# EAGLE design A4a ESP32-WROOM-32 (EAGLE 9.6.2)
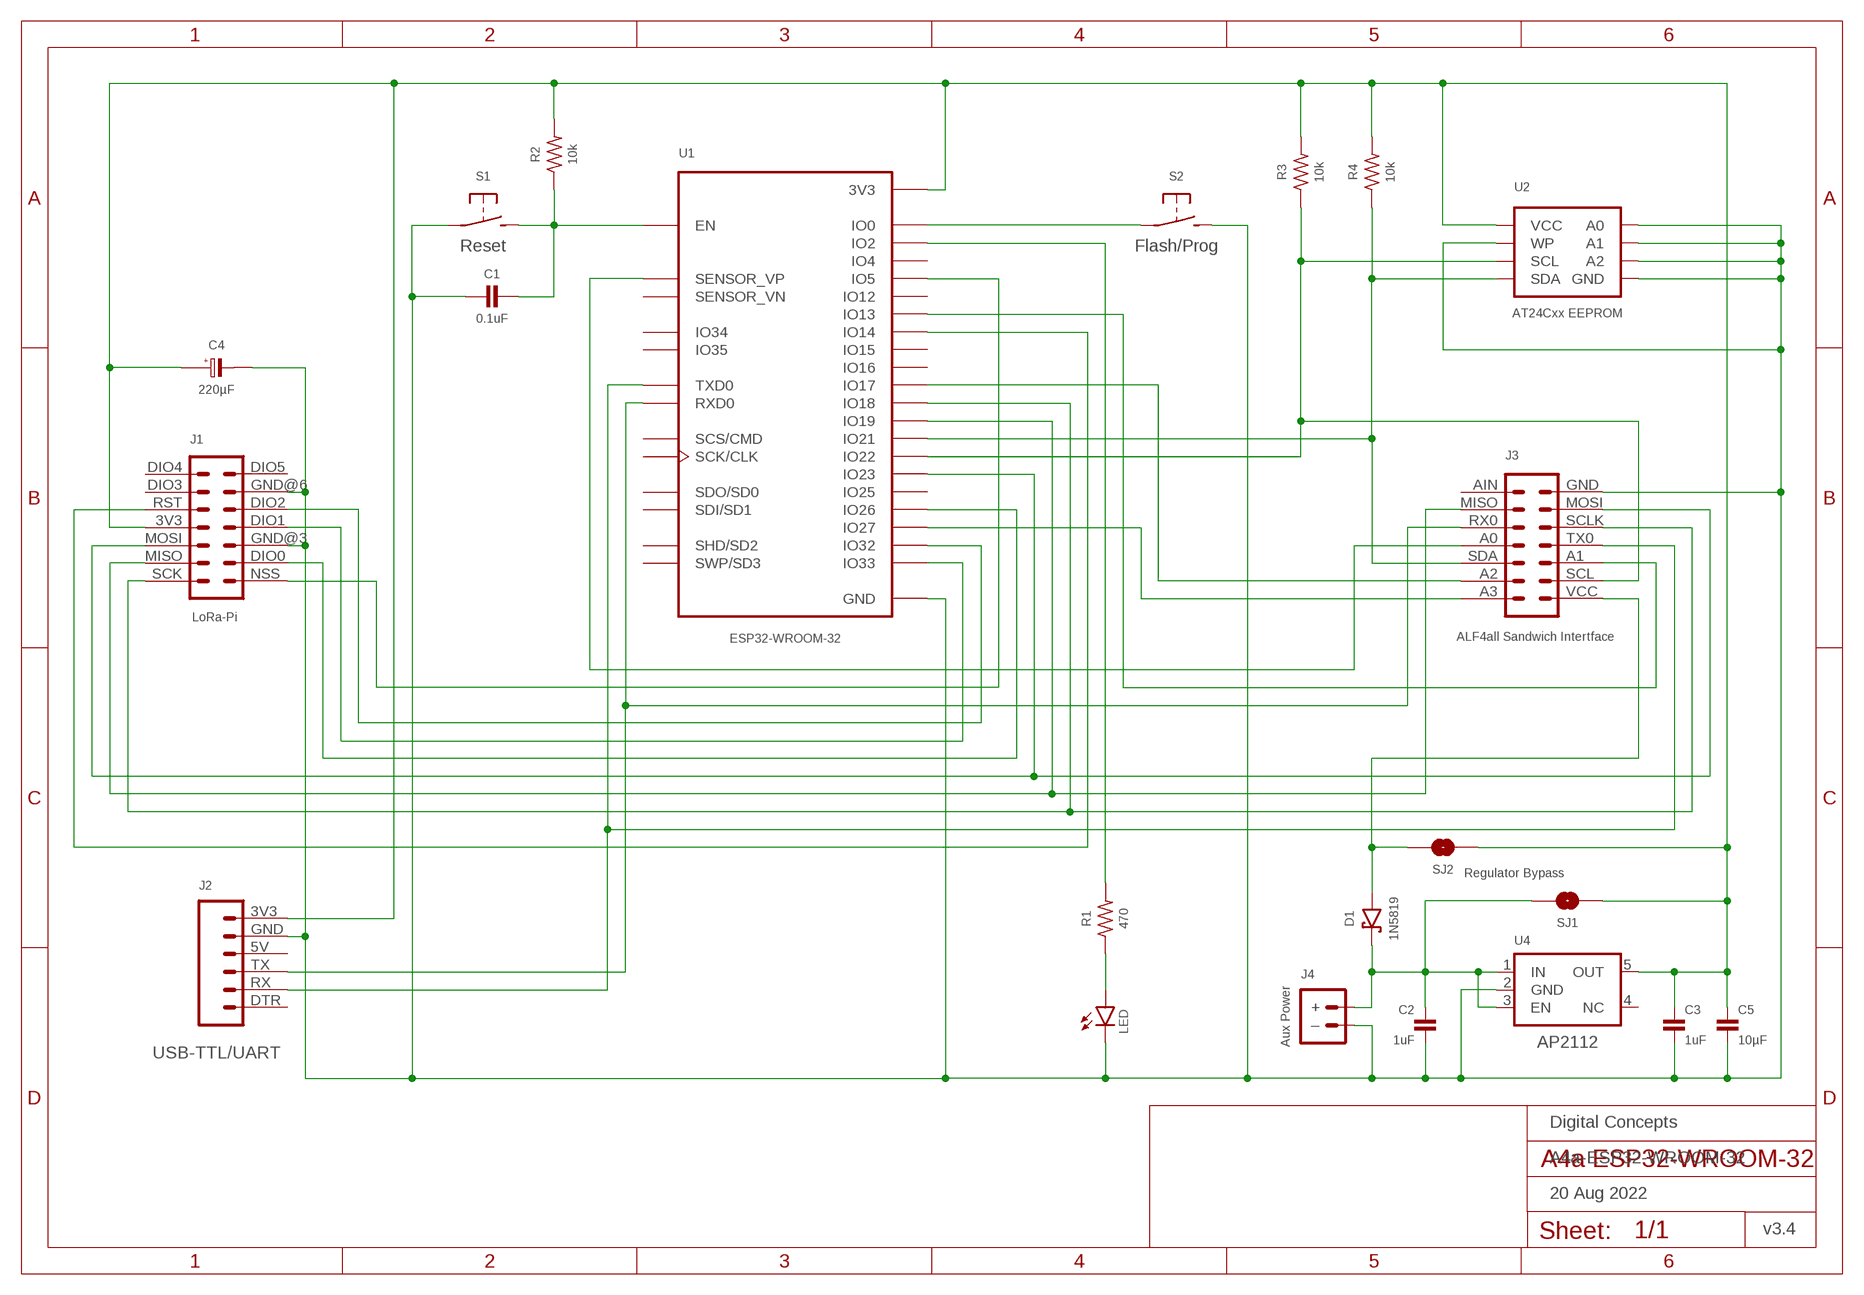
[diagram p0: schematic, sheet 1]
FRAME1 (A4L-LOC): DATE: 20 Aug 2022; OWNER: Digital Concepts; TITLE: A4a-ESP32-WROOM-32; VERSION: v3.4

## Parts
C1  0.1uF  CAPACITOR  [C0805@1]
C2  1uF  CAPACITOR-0805  [C0805]
C3  1uF  CAPACITOR-0805  [C0805]
C4  220µF  CAPACITOR-TANTALUM-3528  [C3528-21]
C5  10µF  CAPACITOR-0805  [C0805]
D1  1N5819  DIODE-SCHOTTKY-1N5819  [SOD-123]
J1  LoRa-Pi  RFM95W-PI-HEADER  [RFM95W-PI]
J2  USB-TTL/UART  HEADER-1X6-UART  [CONN_06-UART]
J3  ALF4all Sandwich Intertface  HEADER-2X7-ALF4ALL-PROCESSOR-B  [CONN_2X7-ALF4ALL-PROCESSOR-B]
J4  Aux Power  JST-PH2.0-2-MALE-HORIZONTALJST-PTH-2  [JST-PH2.0-2-HORIZONTAL]
LED  LEDCHIP-LED0805  [CHIP-LED0805]
R1  470  RESISTORR0805  [R0805]
R2  10k  RESISTORR0805  [R0805]
R3  10k  RESISTORR0805  [R0805]
R4  10k  RESISTORR0805  [R0805]
S1  Reset  SWITCH-MOMENTARY-2-PIN  [SWITCH-2-PAD]
S2  Flash/Prog  SWITCH-MOMENTARY-2-PIN  [SWITCH-2-PAD]
SJ1  Regulator Bypass  SJ  [SJ]
SJ2  SJ  [SJ]
U1  ESP32-WROOM-32  [ESP32-WROOM-32]
U2  AT24Cxx EEPROM  AT24CXX-EEPROM  [SOP-8]
U4  AP2112  REGULATOR-AP2112  [SOT25]

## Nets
GND: C1.2 C2.2 C3.2 C4.2(-) C5.2 J1.GND@3 J1.GND@6 J2.GND J3.GND J4.-(–) LED.C S1.P$1(P) S2.P$2(S) U1.GND@1(GND) U1.GND@15(GND) U1.GND@38(GND) U1.TP(GND) U1.TP@P1(GND) U1.TP@P2(GND) U1.TP@P3(GND) U1.TP@P4(GND) U1.TP@P5(GND) U1.TP@P6(GND) U1.TP@P7(GND) U1.TP@P8(GND) U1.TP@P9(GND) U1.TP@V1(GND) U1.TP@V2(GND) U1.TP@V3(GND) U1.TP@V4(GND) U1.TP@V5(GND) U1.TP@V6(GND) U1.TP@V7(GND) U1.TP@V8(GND) U1.TP@V9(GND) U1.TP@V10(GND) U1.TP@V11(GND) U1.TP@V12(GND) U1.TP@VP5(GND) U2.P$1(A0) U2.P$2(A1) U2.P$3(A2) U2.P$4(GND) U2.P$7(WP) U4.2(GND)
N$1: J1.DIO2 U1.IO32
N$2: J1.NSS U1.IO5
N$3: J1.SCK J3.SCLK U1.IO18
N$4: J1.RST U1.IO14
N$5: J1.MISO J3.MISO U1.IO19
N$6: J1.MOSI J3.MOSI U1.IO23
N$7: LED.A R1.1
N$8: S2.P$1(P) U1.IO0
N$9: J3.A2 U1.IO17
N$10: C2.1 D1.C J4.+ SJ1.1 U4.1(IN) U4.3(EN)
N$11: D1.A J3.VCC SJ2.1
N$12: J3.SCL R3.1 U1.IO22 U2.P$6(SCL)
N$13: C1.1 R2.1 S1.P$2(S) U1.EN
N$14: J3.SDA R4.1 U1.IO21 U2.P$5(SDA)
N$15: J3.A1 U1.IO13
N$16: J2.TX J3.RX0 U1.RXD0
N$17: R1.2 U1.IO2
N$18: J1.DIO0 U1.IO26
N$21: J3.A0 U1.SENSOR_VP
N$22: J3.A3 U1.IO27
N$26: J1.DIO1 U1.IO33
VC: J2.RX J3.TX0 U1.TXD0
VCC: C3.1 C4.1(+) C5.1 J1.3V3 J2.3V3 R2.2 R3.2 R4.2 SJ1.2 SJ2.2 U1.3V3 U2.P$8(VCC) U4.5(OUT)
Unconnected: J1.DIO3 J1.DIO4 J1.DIO5 J2.5V J2.DTR J3.AIN U1.CLK(SCK/CLK) U1.CMD(SCS/CMD) U1.IO4 U1.IO12 U1.IO15 U1.IO16 U1.IO25 U1.IO34 U1.IO35 U1.SD0(SDO/SD0) U1.SD1(SDI/SD1) U1.SD2(SHD/SD2) U1.SD3(SWP/SD3) U1.SENSOR_VN U4.4(NC)

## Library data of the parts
C1 = digitalconcepts:CAPACITOR: 0805 Capacitor
C2 C3 C5 = digitalconcepts:CAPACITOR-0805: 0805 Capacitor
C4 = digitalconcepts:CAPACITOR-TANTALUM-3528: Capacitor Polarised EIA 3528-21 (KEMET B)
D1 = digitalconcepts:DIODE-SCHOTTKY-1N5819: 1N5819 Schottky Diode SOD-123
J1 = digitalconcepts:RFM95W-PI-HEADER: RFM95W LoRa Wireless Transceiver Raspberry Pi Daughter Board
J2 = digitalconcepts:HEADER-1X6-UART: UART 6-Pin Header
J3 = digitalconcepts:HEADER-2X7-ALF4ALL-PROCESSOR-B: ALF4all 'Sandwich' Processor (Bottom) 2x7 Pin Header Header soldered to underside of PCB
J4 = digitalconcepts:JST-PH2.0-2-MALE-HORIZONTAL: PH2.0 2P Right Angle PCB Connector; PROD_ID: CONN-09863; SKU: PRT-09914
LED = digitalconcepts:LED: LED
R1-R4 = digitalconcepts:RESISTOR: Resistor; SPICEPREFIX: R
S1 S2 = digitalconcepts:SWITCH-MOMENTARY-2-PIN: 2 Pin Momentary Switch
SJ1 SJ2 = digitalconcepts:SJ: Solder Jumper
U1 = digitalconcepts:ESP32-WROOM-32: ESP32-WROOM-32 MCU
U2 = digitalconcepts:AT24CXX-EEPROM: AT24Cxx EEPROM SOP-8
U4 = digitalconcepts:REGULATOR-AP2112: Diodes Incorporated LDO Regulator with Enable; OC_FARNELL: unknown; OC_NEWARK: unknown

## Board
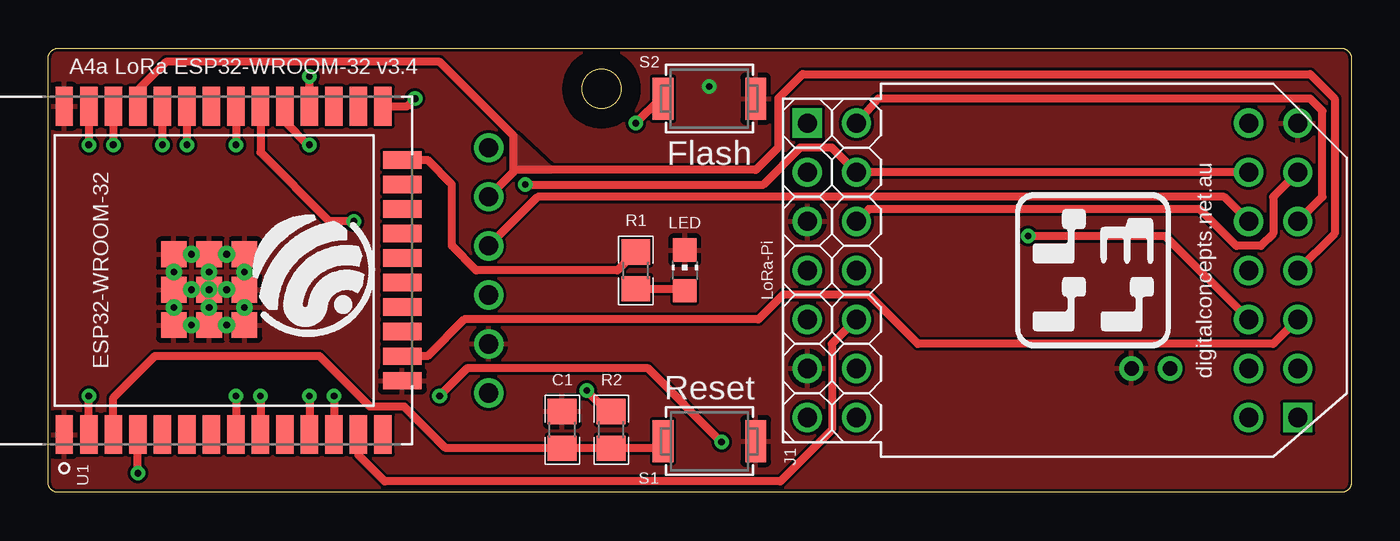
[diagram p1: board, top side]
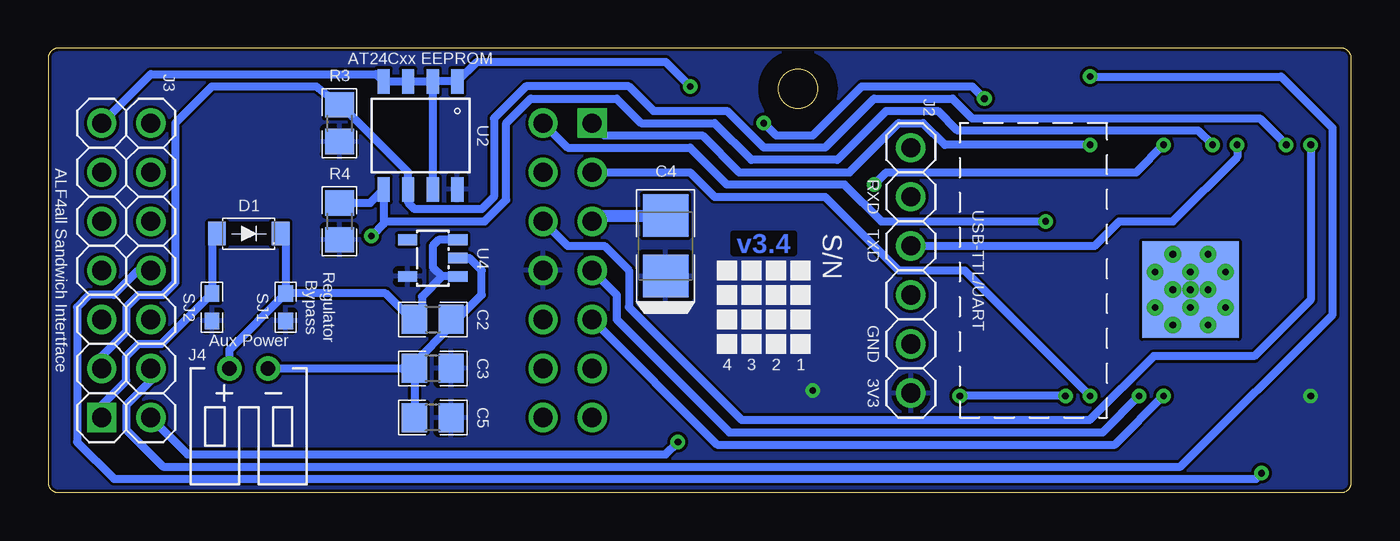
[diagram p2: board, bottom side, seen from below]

Size 67.49 x 23 mm. Coordinates in mm from the lower left corner, seen from the top.
Outline: 88 segments
Outline: circle at 28.65,20.9 radius 1.02
Copper layers (1*16): Top 0.035mm / dielectric 1.5mm / Bottom 0.035mm
Design rules "default *": minimum track width 6mil, minimum drill 0.35mm, track to track 6mil, track to pad 6mil, pad to pad 6mil, via to via 6mil, smd to smd 6mil, copper to edge 6mil, drill to drill 6mil, minimum pad ring 10mil, minimum via ring 8mil, stop-mask expansion 4mil, vias tented up to drill 0mil, thermal gap 10mil

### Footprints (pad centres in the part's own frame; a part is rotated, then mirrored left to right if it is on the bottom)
C0805@1 = smd 1.3 x 1.5: 1 -0.95,0; 2 0.95,0
C0805 = smd 1.3 x 1.5: 1 -0.95,0; 2 0.95,0
C3528-21 = smd 2.21 x 2.35: 1 -1.565,0; 2 1.565,0
SOD-123 = smd 0.91 x 1.22: A -1.65,0; C 1.65,0
RFM95W-PI = drill 1 pad 1.524: 3V3 7.62,2.54; DIO0 2.54,0; DIO1 7.62,0; DIO2 10.16,0; DIO3 12.7,2.54; DIO4 15.24,2.54; DIO5 15.24,0; GND@3 5.08,0; GND@6 12.7,0; MISO 2.54,2.54; MOSI 5.08,2.54; RST 10.16,2.54; SCK 0,2.54 | drill 1 pad 1.524 square: NSS 0,0
CONN_06-UART = drill 1 pad 1.524: 3V3 12.7,0; 5V 7.62,0; DTR 0,0; GND 10.16,0; RX 2.54,0; TX 5.08,0
CONN_2X7-ALF4ALL-PROCESSOR-B = drill 1 pad 1.524: A0 7.62,2.54; A1 5.08,0; A2 2.54,2.54; A3 0,2.54; AIN 15.24,2.54; GND 15.24,0; MISO 12.7,2.54; MOSI 12.7,0; RX0 10.16,2.54; SCL 2.54,0; SCLK 10.16,0; SDA 5.08,2.54; TX0 7.62,0 | drill 1 pad 1.524 square: VCC 0,0
JST-PH2.0-2-HORIZONTAL = drill 0.75: + 1,0; - -1,0
CHIP-LED0805 = smd 1.2 x 1.2: A 0,-1.05; C 0,1.05
R0805 = smd 1.3 x 1.5: 1 -0.95,0; 2 0.95,0
SWITCH-2-PAD = smd 1.067 x 2.184: P$1 -2.4,0; P$2 2.4,0
SJ = smd 0.864 x 0.762: 1 -0.711,0; 2 0.711,0
ESP32-WROOM-32 = smd 2 x 0.9: 3V3 -8.5,6.74; EN -8.5,5.47; GND@1 -8.5,8.01; GND@38 8.5,8.01; IO0 8.5,-8.5; IO4 8.5,-7.23; IO5 8.5,-3.42; IO12 -8.5,-8.5; IO14 -8.5,-7.23; IO16 8.5,-5.96; IO17 8.5,-4.69; IO18 8.5,-2.15; IO19 8.5,-0.88; IO21 8.5,1.66; IO22 8.5,5.47; IO23 8.5,6.74; IO25 -8.5,-3.42; IO26 -8.5,-4.69; IO27 -8.5,-5.96; IO32 -8.5,-0.88; IO33 -8.5,-2.15; IO34 -8.5,1.66; IO35 -8.5,0.39; NC 8.5,0.39; RXD0 8.5,2.93; SENSOR_VN -8.5,2.93; SENSOR_VP -8.5,4.2; TXD0 8.5,4.2 | smd 0.9 x 2: CLK 0.635,-9.5; CMD -0.635,-9.5; GND@15 -5.715,-9.5; IO2 5.715,-9.5; IO13 -4.445,-9.5; IO15 4.445,-9.5; SD0 1.905,-9.5; SD1 3.175,-9.5; SD2 -3.175,-9.5; SD3 -1.905,-9.5 | smd 5 x 5 bottom: TP -1,0.51 | smd 1.33 x 1.33: TP@P1 -2.835,2.335; TP@P2 -1,2.335; TP@P3 0.835,2.335; TP@P4 -2.835,0.51; TP@P5 -1,0.51; TP@P6 0.835,0.51; TP@P7 -2.835,-1.325; TP@P8 -1,-1.325; TP@P9 0.835,-1.325 | drill 0.35 pad 0.406: TP@V1 -1.917,2.335; TP@V2 -0.083,2.335; TP@V3 -2.835,1.423; TP@V4 -1,1.423; TP@V5 0.835,1.423; TP@V6 -1.917,0.51; TP@V7 -0.083,0.51; TP@V8 -2.835,-0.403; TP@V9 -1,-0.403; TP@V10 0.835,-0.403; TP@V11 -1.917,-1.325; TP@V12 -0.083,-1.325; TP@VP5 -1,0.51
SOP-8 = smd 0.635 x 1.27: P$1 -1.905,-2.794; P$2 -0.635,-2.794; P$3 0.635,-2.794; P$4 1.905,-2.794; P$5 1.905,2.794; P$6 0.635,2.794; P$7 -0.635,2.794; P$8 -1.905,2.794
SOT25 = smd 0.55 x 1: 1 -0.95,-1.3; 2 0,-1.3; 3 0.95,-1.3; 4 0.95,1.3; 5 -0.95,1.3

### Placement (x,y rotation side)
C1  26.62,3.25 90 top
C2  47.57,8.96 0 bottom
C3  47.57,6.42 180 bottom
C4  35.51,12.77 90 bottom
C5  47.57,3.88 180 bottom
D1  57.1,13.41 0 bottom
J1  39.32,19.12 270 top
J2  22.81,17.85 270 bottom
J3  64.72,3.88 90 top
J4  57.1,6.42 180 bottom
LED  32.97,11.5 0 top
R1  30.43,11.5 90 top
R2  29.16,3.25 90 top
R3  52.4,19.12 270 bottom
R4  52.4,14.04 270 bottom
S1  34.24,2.66 180 top
S2  34.24,20.39 0 top
SJ1  55.19,9.6 270 bottom
SJ2  59,9.6 270 bottom
U1  8.84,11.5 90 top
U2  48.21,18.49 180 bottom
U4  47.57,12.14 90 bottom

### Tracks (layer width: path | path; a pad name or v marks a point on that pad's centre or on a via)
$X1
  cutout Top: 28.65,22.93 arc180 28.65,18.87 arc180
$X2
  cutout Bottom: 28.65,22.93 arc180 28.65,18.87 arc180
GND  (via drill 0.35)
  Bottom 0.406: U2.P$2 U2.P$3 U2.P$4 50.5,21.66 62.18,21.66 J3.GND | U2.P$2 U2.P$7 | J4.- C3.2 | U2.P$2 U2.P$1 45.29,22.3 35.51,22.3 v34.24,21.03 | 46.47,9.11 C2.2 | C3.2 48.52,6.73 46.62,8.63 C2.2 | C3.2 C5.2 | C2.2 46.3,8.96 45.03,10.23 45.03,11.5 45.67,12.14 U4.2
  Bottom 0.61: J1.GND@3 39.02,14.34 C4.2
  pour Top (rank 3): -1.32,24.2 68.53,24.2 68.53,-1.2 -1.32,-1.2
N$1  (via drill 0.35)
  Top 0.406: v9.72,5 U1.IO32
  Bottom 0.406: J1.DIO2 32.84,2.48 12.24,2.48 v9.72,5
N$2  (via drill 0.35)
  Top 0.406: U1.IO5 12.26,19.19 13.49,17.96 v13.53,18
  Bottom 0.406: J1.NSS 38.68,18.49 33.6,18.49 31.7,16.58 25.98,16.58 23.44,19.12 22.17,19.12 21.05,18 v13.53,18
N$3  (via drill 0.35)
  Top 0.406: J3.SCLK 65.99,15.31 65.99,19.76 65.35,20.39 42.98,20.39 J1.SCK | U1.IO18 10.99,17.61 14.55,14.04 v15.82,14.04
  Bottom 0.406: J1.SCK 40.59,17.85 34.24,17.85 32.33,15.95 26.24,15.95 24.33,14.04 v15.82,14.04
N$4
  Top 0.406: J1.RST 40.59,7.69 40.59,3.25 37.92,0.58 17.43,0.58 16.07,1.94 U1.IO14
N$5  (via drill 0.35)
  Top 0.406: J3.MISO J1.MISO 40.59,17.85 38.94,17.85 37.03,15.95 v24.71,15.95 | U1.IO19 v9.72,18
  Bottom 0.406: v9.72,18 11.14,16.58 24.08,16.58 v24.71,15.95
N$6  (via drill 0.35)
  Top 0.406: J3.MOSI 63.45,15.31 63.45,13.41 62.81,12.77 61.54,12.77 59.64,14.68 42.49,14.68 J1.MOSI | U1.IO23 v2.1,18
  Bottom 0.406: J1.MOSI 40.59,12.77 38.68,12.77 37.41,11.5 37.41,9.6 31.57,3.75 13.54,3.75 10.24,7.06 5.02,7.06 2.1,9.98 v2.1,18
N$7
  Top 0.406: R1.1 32.87,10.55 LED.A
N$8  (via drill 0.35)
  Top 0.406: U1.IO0 18.61,20 v19,20.39 | S2.P$1 31.7,20.39 v30.43,19.12
  Bottom 0.406: v19,20.39 19.63,21.03 25.35,21.03 27.89,18.49 29.79,18.49 v30.43,19.12
N$9  (via drill 0.35)
  Top 0.406: U1.IO17 v13.53,21.53
  Bottom 0.406: J3.A2 62.18,5.79 63.45,4.52 63.45,3.25 61.54,1.34 8.84,1.34 0.97,9.22 0.97,18.87 3.63,21.53 v13.53,21.53
N$10
  Bottom 0.406: SJ1.1 50.02,10.31 48.67,8.96 C2.1 48.13,9.35 48.13,10.15 47.09,11.19 | J4.+ 58.1,7.4 SJ1.1 | D1.C 55.19,13.15 SJ1.1 | U4.1 47.09,11.19 | U4.3 47.26,13.09 47.57,12.77 47.57,11.67 47.09,11.19
  pour Bottom: 47.57,11.67 47.57,10.7 47.09,11.19
N$11
  Bottom 0.406: J3.VCC 64.72,4.52 63.45,5.79 63.45,7.06 62.81,7.69 61.62,7.69 SJ2.1 59,13.15 D1.A
N$12  (via drill 0.35)
  Top 0.406: U1.IO22 v3.37,18
  Bottom 0.406: v3.37,18 4.74,19.38 19.63,19.38 20.65,20.39 24.71,20.39 27.25,17.85 30.43,17.85 32.33,19.76 36.14,19.76 37.41,21.03 42.75,21.03 44.4,19.38 44.4,15.31 45.03,14.68 48.51,14.68 48.84,15.01 U2.P$6 48.84,16.58 52.33,20.07 R3.1 53.61,21.03 59,21.03 60.91,19.12 60.91,10.87 61.54,10.23 62.81,10.23 63.45,9.6 63.45,8.33 64.72,7.06 J3.SCL
N$13
  Top 0.406: U1.EN 3.37,4.91 5.52,7.06 14.05,7.06 16.66,4.44 18.44,4.44 20.58,2.3 C1.1 R2.1 31.48,2.3 S1.P$2
N$14  (via drill 0.35)
  Top 0.406: U1.IO21 v7.18,18 | v50.75,13.28 57.86,13.28 J3.SDA
  Bottom 0.406: v7.18,18 7.92,18.74 20.4,18.74 21.41,19.76 24.08,19.76 26.62,17.22 31.06,17.22 32.97,19.12 36.78,19.12 38.05,20.39 42.49,20.39 43.76,19.12 43.76,15.16 44.88,14.04 49.99,14.04 v50.75,13.28 50.11,13.91 U2.P$5 50.82,14.99 R4.1
N$15
  Top 0.406: J3.A1 63.45,7.69 45.03,7.69 42.49,10.23 38.05,10.23 36.78,8.96 21.54,8.96 19.63,7.06 U1.IO13
N$16  (via drill 0.35)
  Top 0.406: J3.RX0 60.91,15.31 25.35,15.31 J2.TX | U1.RXD0 v5.91,18
  Bottom 0.406: v5.91,18 5.91,17.37 9.23,14.04 12.01,14.04 13.28,12.77 J2.TX
N$17
  Top 0.406: U1.IO2 19.63,17.22 20.9,15.95 20.9,12.77 22.17,11.5 29.48,11.5 R1.2
N$18  (via drill 0.35)
  Top 0.406: v13.53,5 U1.IO26
  Bottom 0.406: J1.DIO0 34.24,16.58 32.97,15.31 27.25,15.31 23.44,11.5 20.03,11.5 v13.53,5
N$21  (via drill 0.35)
  Top 0.406: v4.64,1 U1.SENSOR_VP
  Bottom 0.406: J3.A0 62.83,11.5 64.1,10.23 65.35,10.23 65.99,9.6 65.99,2.61 64.08,0.71 4.93,0.71 v4.64,1
N$22  (via drill 0.35)
  Top 0.406: v34.87,2.61 31.06,6.42 21.69,6.42 v20.27,5 | v14.8,5 U1.IO27
  Bottom 0.406: v34.87,2.61 35.51,1.98 60.27,1.98 J3.A3 | v14.8,5 v20.27,5
N$26  (via drill 0.35)
  Top 0.406: v10.99,5 U1.IO33
  Bottom 0.406: J1.DIO1 38.05,10.23 38.05,8.96 32.21,3.12 12.87,3.12 v10.99,5
VC
  Top 0.406: J3.TX0 66.62,13.41 66.62,20.39 65.35,21.66 39.07,21.66 37.8,20.39 37.8,17.85 36.65,16.71 24.08,16.71 | 24.08,16.71 24.08,18.49 20.27,22.3 6.1,22.3 4.64,20.84 U1.TXD0 | 24.08,16.71 24.08,16.58 J2.RX
  pour Top: 24.08,18.49 24.08,16.71 25.98,16.71
VCC  (via drill 0.35)
  Top 0.406: U1.3V3 v2.1,5 | v27.89,5.28 28.97,4.2 R2.2
  pour Bottom (rank 3): -0.69,23.57 67.89,23.57 67.89,-0.56 -0.69,-0.56

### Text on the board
Bottom: v3.4
tPlace: A4a LoRa ESP32-WROOM-32 v3.4 | digitalconcepts.net.au
bPlace: S/N | 1 | 2 | 3 | 4
bNames: RXD | TXD | Regulator / Bypass | GND | 3V3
